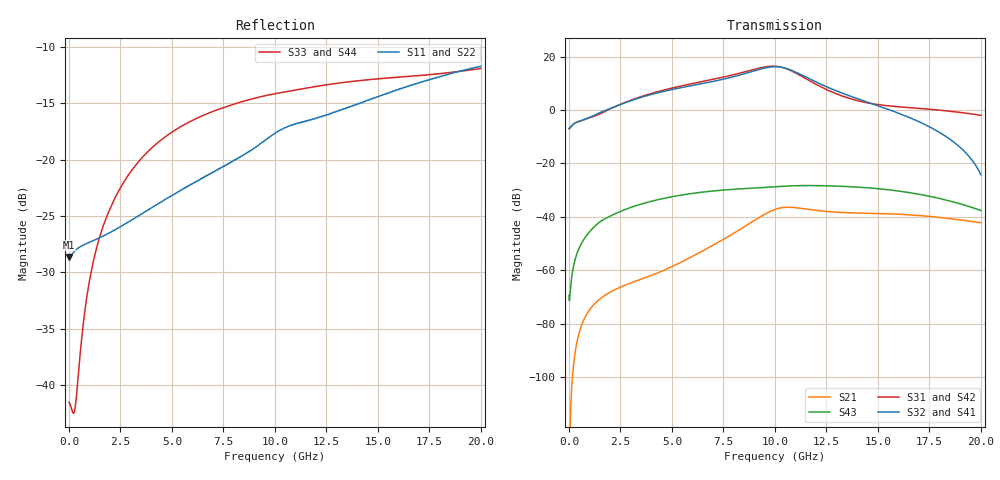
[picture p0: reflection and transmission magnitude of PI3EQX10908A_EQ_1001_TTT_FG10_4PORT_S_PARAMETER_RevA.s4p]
! NPort=4 DATA=2000 NOISE=0 GROUPDELAY=0 COMPLEX_DATAFORMAT=POLAR
! NumOfBlock=1 NumOfParam=0
! .MODEL Smodel S TSTONEFILE=PI3EQX10908A_EQ_1001_TTT_FG10_4PORT_S_PARAMETER_RevA.s4p TYPE=S
!  -- The above .MODEL line can be used for the S element in the netlist.
! The s parameter is extracted from the linear redriver, it is not bi-directional; only s(4,1)s(4,2) and s(3,1)s(3,2)
! should be the insertion loss
!Port definition:
!Port1 = input+
!Port2 = input-
!Port3 = output+
!Port4 = output-
# Hz S MA R  50
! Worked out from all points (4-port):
!   2000 points, 10 MHz to 20 GHz, reference 50 ohm
!   strongest paths, dB at 10 MHz, 5.01 GHz, 10.01 GHz, 15.01 GHz, 20 GHz:
!     S32: -6.9, 7.7, 16.2, 1.6, -24.2
!     S41: -6.9, 7.7, 16.2, 1.6, -24.2
!     S31: -6.9, 8.3, 16.4, 2.0, -2.0
!     S42: -6.9, 8.3, 16.4, 2.0, -2.0
!     S43: -69.4, -32.4, -28.7, -29.5, -37.6
!     S21: -127.2, -58.6, -37.2, -38.7, -42.2
!   lowest |S11| = -28.6 dB at 10 MHz (marker M1), VSWR 1.08, Z = 46.4 - j0.024 ohm
!   |S11| at or under -10 dB: start of sweep to end of sweep
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1e7  0.03701 -179.6  4.34e-07 14.5  0 0.0  0 0.0
     4.34e-07 14.5  0.03701 -179.6  0 0.0  0 0.0
     0.4507 1.1  0.4507 -178.9  0.008374 26.0  0.00034 -27.1
     0.4507 -178.9  0.4507 1.1  0.00034 -27.1  0.008374 26.0
6.97e9  0.08789 -119.2  0.002913 133.4  4.984e-07 61.4  2.489e-07 135.4
        0.002912 133.4  0.08792 -119.2  2.489e-07 135.4  4.984e-07 61.4
        3.743 -52.5  3.424 120.9  0.1634 10.0  0.03045 13.9
        3.424 120.9  3.743 -52.5  0.03045 13.9  0.1634 10.0
9.25e9  0.1171 -111.4  0.009803 111.6  2.814e-06 16.8  1.756e-06 116.3
        0.009804 111.7  0.1171 -111.4  1.756e-06 116.3  2.815e-06 16.7
        6.115 -111.8  5.788 62.6  0.1896 -7.5  0.0351 -9.4
        5.788 62.7  6.115 -111.8  0.0351 -9.4  0.1896 -7.5
1.038e10  0.137 -111.9  0.01492 74.1  4.444e-06 -17.4  4.743e-06 81.6
          0.01492 74.1  0.137 -111.9  4.744e-06 81.6  4.445e-06 -17.4
          6.269 -163.7  6.265 9.7  0.1989 -15.0  0.03742 -20.8
          6.265 9.7  6.269 -163.7  0.03742 -20.8  0.1989 -15.0
1.144e10  0.1477 -113.3  0.01415 42.8  5.061e-06 -27.0  7.819e-06 44.9
          0.01414 42.8  0.1477 -113.3  7.821e-06 44.9  5.061e-06 -27.0
          4 155.8  4.269 -34.3  0.207 -21.2  0.03856 -33.8
          4.269 -34.2  3.999 155.8  0.03856 -33.8  0.207 -21.2
1.361e10  0.1717 -111.7  0.01194 14.8  1.364e-05 -36.6  1.658e-05 -4.8
          0.01193 14.8  0.1718 -111.7  1.659e-05 -4.8  1.364e-05 -36.6
          1.656 126.8  1.854 -81.7  0.2216 -32.5  0.03682 -60.1
          1.854 -81.7  1.656 126.8  0.03682 -60.1  0.2216 -32.5
2e10  0.2599 -114.7  0.007803 -40.4  8.951e-05 -147.8  7.215e-05 -138.5
      0.007797 -40.3  0.26 -114.7  7.216e-05 -138.5  8.95e-05 -147.8
      0.7972 55.5  0.06146 171.4  0.2539 -52.2  0.01317 -136.6
      0.06167 171.9  0.7977 55.5  0.01316 -136.6  0.2539 -52.2
